// Version 2.0, 05.09.99: Änderungen:
// Umstrukturierungen und Bearbeitungzeitoptimierung,
// Quittierung von DB71-Aufträgen sofort
// FC90_3

FUNCTION FC 90 : VOID
TITLE = ANSTEUERUNG QUIT_WZV
VERSION : 2.0

BEGIN
      U     E      3.7; // Taste Reset
      FP    M    190.1;
      =     M    190.2; // Flanke Taste Reset
	U	DB71.DBX	0.1;
	SPBN  SS1
; // SS2 Be/Entladen aktiv ? nein ->
      U     DB71.DBX   34.0; // Beladen aktiv
//    U     M    190.0; // Flanke beladen Magazin beendet
      S     DB90.DBX    0.0; // ASS 1:Quittung WZ beladen beendet
	R	DB71.DBX   34.0; // Beladen aktiv
NETWORK
TITLE =Abbruch/Reset Werkzeug beladen Magazin
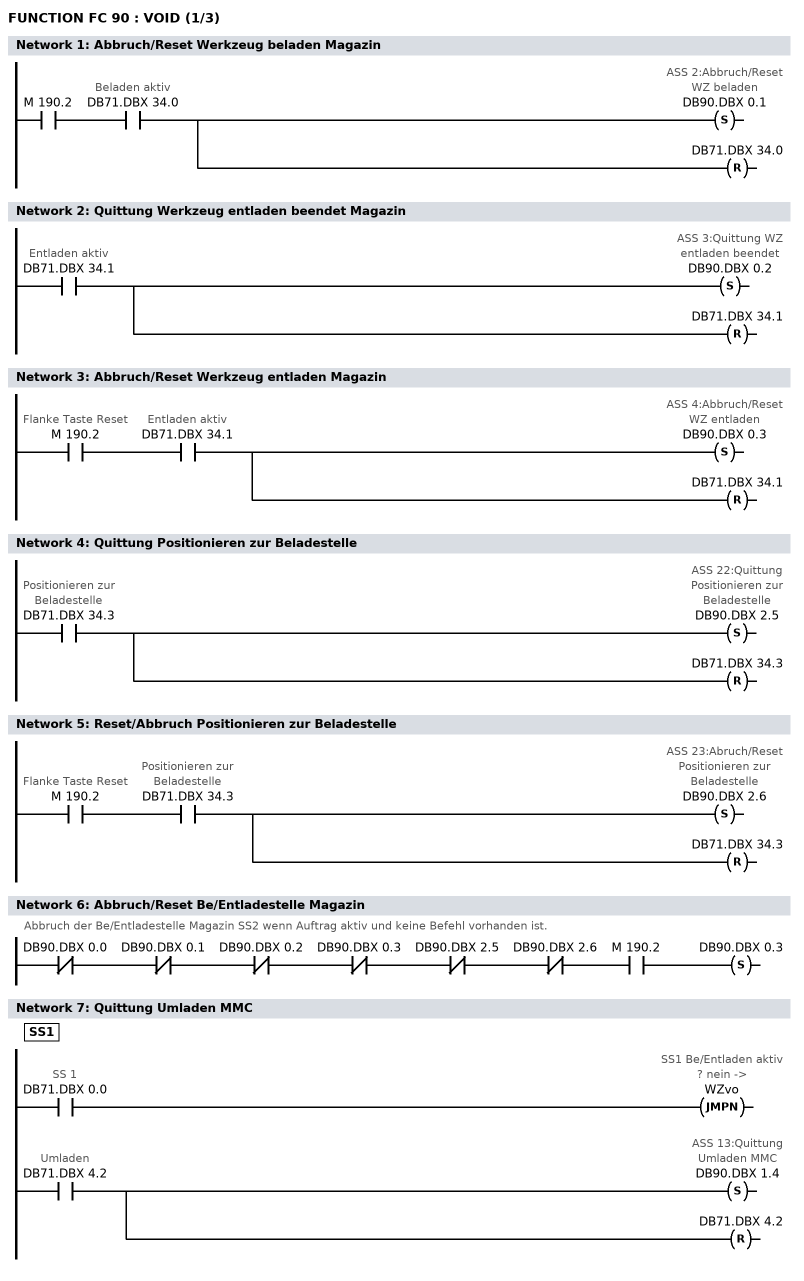
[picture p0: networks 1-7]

      U     M    190.2;
      U     DB71.DBX   34.0; // Beladen aktiv
      S     DB90.DBX    0.1; // ASS 2:Abbruch/Reset WZ beladen
	R	DB71.DBX   34.0;
NETWORK
TITLE =Quittung Werkzeug entladen beendet Magazin

      U     DB71.DBX   34.1; // Entladen aktiv
//    U     M    190.3; // Flanke entladen Magazin beendet
      S     DB90.DBX    0.2; // ASS 3:Quittung WZ entladen beendet
	R	DB71.DBX	34.1;
NETWORK
TITLE =Abbruch/Reset Werkzeug entladen Magazin

      U     M    190.2; // Flanke Taste Reset
      U     DB71.DBX   34.1; // Entladen aktiv
      S     DB90.DBX    0.3; // ASS 4:Abbruch/Reset WZ entladen
	R	DB71.DBX   34.1;

NETWORK
TITLE =Quittung Positionieren zur Beladestelle

      U     DB71.DBX   34.3;  // Positionieren zur Beladestelle
//    U     M    193.2; // Positionieren beendet
      S     DB90.DBX    2.5; // ASS 22:Quittung Positionieren zur Beladestelle
	R	DB71.DBX   34.3;
NETWORK
TITLE =Reset/Abbruch Positionieren zur Beladestelle

      U     M    190.2; // Flanke Taste Reset
      U     DB71.DBX   34.3; // Positionieren zur Beladestelle
      S     DB90.DBX    2.6; // ASS 23:Abruch/Reset Positionieren zur Beladestelle
	R	DB71.DBX   34.3;
NETWORK
TITLE =Abbruch/Reset Be/Entladestelle Magazin
//Abbruch der Be/Entladestelle Magazin SS2 wenn Auftrag aktiv und keine Befehl vorhanden ist.

      UN    DB90.DBX    0.0;
      UN    DB90.DBX    0.1;
      UN    DB90.DBX    0.2;
	UN	DB90.DBX	0.3;
	UN    DB90.DBX    2.5;
      UN	DB90.DBX	2.6;
      U     M 	190.2;
      S     DB90.DBX    0.3;
NETWORK
TITLE =Quittung Umladen MMC

SS1:  U     DB71.DBX    0.0; // SS 1
	SPBN	WZvo;	// SS1 Be/Entladen aktiv ? nein ->
      U     DB71.DBX    4.2; // Umladen
      S     DB90.DBX    1.4; // ASS 13:Quittung Umladen MMC
	R     DB71.DBX    4.2;
NETWORK
TITLE =Quittung Wechsel vorbereiten beendet
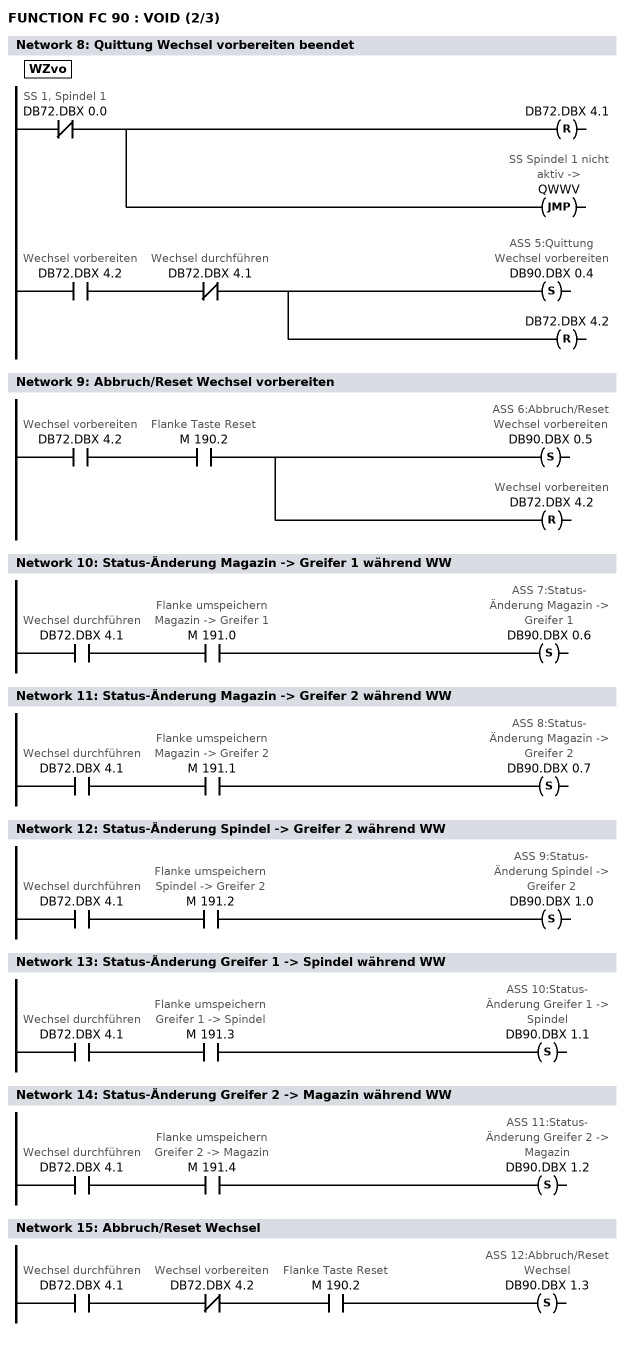
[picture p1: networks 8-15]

WZvo: UN	DB72.DBX	0.0; // SS 1, Spindel 1
	R	DB72.DBX	4.1;
      SPB  QWWV; // SS Spindel 1 nicht aktiv ->
	U     DB72.DBX    4.2; // Wechsel vorbereiten
      UN    DB72.DBX    4.1; // Wechsel durchführen
//    U     M    190.4; // Flanke Wechsel vorbereitet beendet
      S     DB90.DBX    0.4; // ASS 5:Quittung Wechsel vorbereiten
      R	DB72.DBX	4.2;
NETWORK
TITLE =Abbruch/Reset Wechsel vorbereiten

      U     DB72.DBX    4.2; // Wechsel vorbereiten
      U     M    190.2; // Flanke Taste Reset
      S     DB90.DBX    0.5; // ASS 6:Abbruch/Reset Wechsel vorbereiten
      R     DB72.DBX    4.2; // Wechsel vorbereiten
NETWORK
TITLE =Status-Änderung Magazin -> Greifer 1 während WW

      U     DB72.DBX    4.1; // Wechsel durchführen
      U     M    191.0; // Flanke umspeichern Magazin -> Greifer 1
      S     DB90.DBX    0.6; // ASS 7:Status-Änderung Magazin -> Greifer 1
NETWORK
TITLE =Status-Änderung Magazin -> Greifer 2 während WW

      U     DB72.DBX    4.1; // Wechsel durchführen
      U     M    191.1; // Flanke umspeichern Magazin -> Greifer 2
      S     DB90.DBX    0.7; // ASS 8:Status-Änderung Magazin -> Greifer 2
NETWORK
TITLE =Status-Änderung Spindel -> Greifer 2 während WW

      U     DB72.DBX    4.1; // Wechsel durchführen
      U     M    191.2; // Flanke umspeichern Spindel -> Greifer 2
      S     DB90.DBX    1.0; // ASS 9:Status-Änderung Spindel -> Greifer 2
NETWORK
TITLE =Status-Änderung Greifer 1 -> Spindel während WW

      U     DB72.DBX    4.1; // Wechsel durchführen
      U     M    191.3; // Flanke umspeichern Greifer 1 -> Spindel
      S     DB90.DBX    1.1; // ASS 10:Status-Änderung Greifer 1 -> Spindel
NETWORK
TITLE =Status-Änderung Greifer 2 -> Magazin während WW

      U     DB72.DBX    4.1; // Wechsel durchführen
      U     M    191.4; // Flanke umspeichern Greifer 2 -> Magazin
      S     DB90.DBX    1.2; // ASS 11:Status-Änderung Greifer 2 -> Magazin
NETWORK
TITLE =Abbruch/Reset Wechsel

      U     DB72.DBX    4.1; // Wechsel durchführen
      UN    DB72.DBX    4.2; // Wechsel vorbereiten
      U     M    190.2; // Flanke Taste Reset
      S     DB90.DBX    1.3; // ASS 12:Abbruch/Reset Wechsel
NETWORK
TITLE =Abbruch/Reset Spindel-SS
//Abbruch der Spindel-SS1 wenn Auftrag aktiv und keine Befehl vorhanden ist.
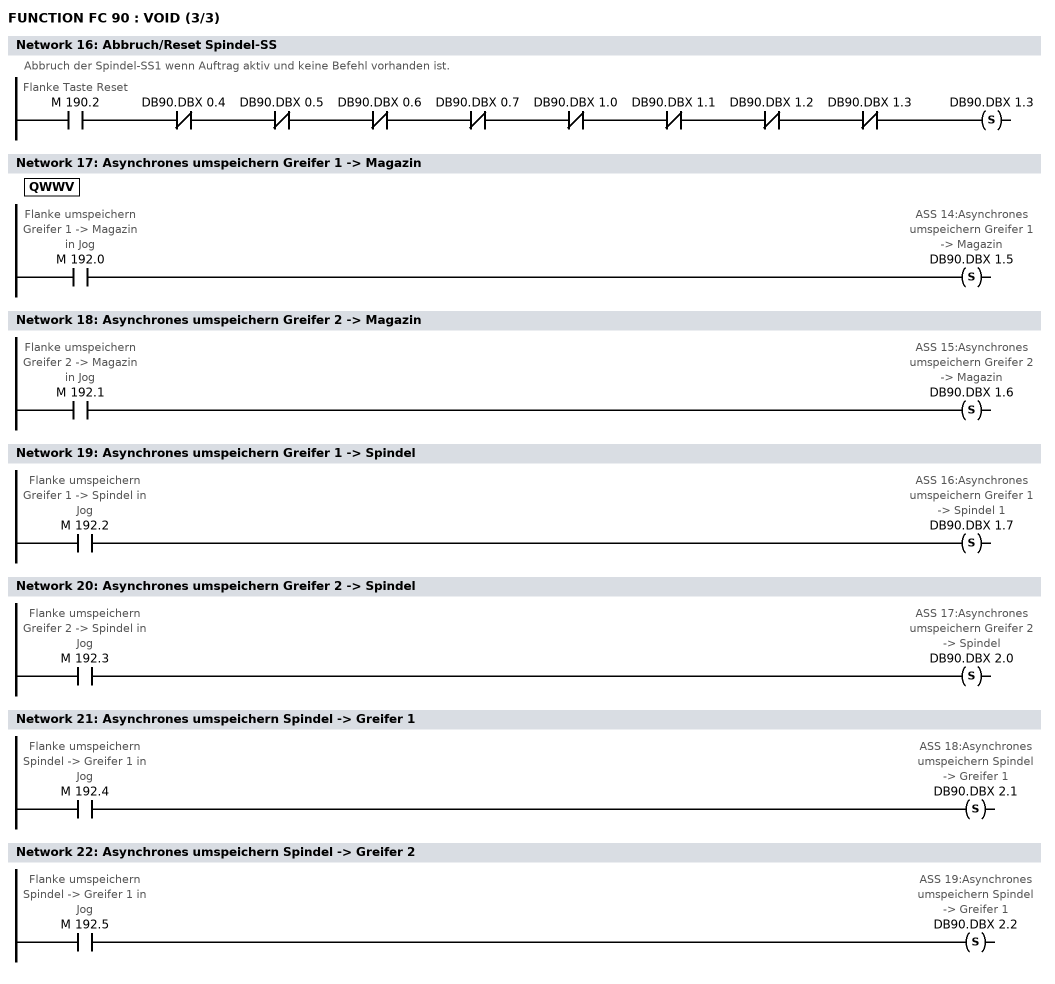
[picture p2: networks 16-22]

	U	M 	190.2; // Flanke Taste Reset
	UN	DB90.DBX	0.4;
	UN	DB90.DBX	0.5;
	UN	DB90.DBX	0.6;
	UN	DB90.DBX	0.7;
	UN	DB90.DBX	1.0;
      UN    DB90.DBX    1.1;
	UN	DB90.DBX	1.2;
	UN	DB90.DBX	1.3;
      S     DB90.DBX    1.3;

NETWORK
TITLE =Asynchrones umspeichern Greifer 1 -> Magazin

QWWV: U     M    192.0; // Flanke umspeichern Greifer 1 -> Magazin in Jog
      S     DB90.DBX    1.5; // ASS 14:Asynchrones umspeichern Greifer 1 -> Magazin
NETWORK
TITLE =Asynchrones umspeichern Greifer 2 -> Magazin

      U     M    192.1; // Flanke umspeichern Greifer 2 -> Magazin in Jog
      S     DB90.DBX    1.6; // ASS 15:Asynchrones umspeichern Greifer 2 -> Magazin
NETWORK
TITLE =Asynchrones umspeichern Greifer 1 -> Spindel

      U     M    192.2; // Flanke umspeichern Greifer 1 -> Spindel in Jog
      S     DB90.DBX    1.7; // ASS 16:Asynchrones umspeichern Greifer 1 -> Spindel 1
NETWORK
TITLE =Asynchrones umspeichern Greifer 2 -> Spindel

      U     M    192.3; // Flanke umspeichern Greifer 2 -> Spindel in Jog
      S     DB90.DBX    2.0; // ASS 17:Asynchrones umspeichern Greifer 2 -> Spindel
NETWORK
TITLE =Asynchrones umspeichern Spindel -> Greifer 1

      U     M    192.4; // Flanke umspeichern Spindel -> Greifer 1 in Jog
      S     DB90.DBX    2.1; // ASS 18:Asynchrones umspeichern Spindel -> Greifer 1
NETWORK
TITLE =Asynchrones umspeichern Spindel -> Greifer 2

      U     M    192.5; // Flanke umspeichern Spindel -> Greifer 1 in Jog
      S     DB90.DBX    2.2; // ASS 19:Asynchrones umspeichern Spindel -> Greifer 1
NETWORK
TITLE =Änderung Istposition
// In MW180 steht die aktuelle Istposition der Wechselstelle in Format Int (ist
// vom Anwender zu versorgen).
      L     DB90.DBW   10; // Istposition alt
      L     MW   180; // Istposition neu
      T     DB90.DBW   10;
      <>I   ;
      S     DB90.DBX    2.3; // ASS 20: Änderung Istposition Magazin
NETWORK
TITLE =Fehlerbit löschen

      U     M    192.7; // Taste Fehler löschen
      R     DB90.DBX    4.0; // Fehler Quittung FC 8
NETWORK
TITLE =Aufruf FB 90
// Aufruf nur wenn QUIT_1 (FB90, DB90) bereits übersetzt wurde.
      CALL FB    90 , DB    90 ;

END_FUNCTION

